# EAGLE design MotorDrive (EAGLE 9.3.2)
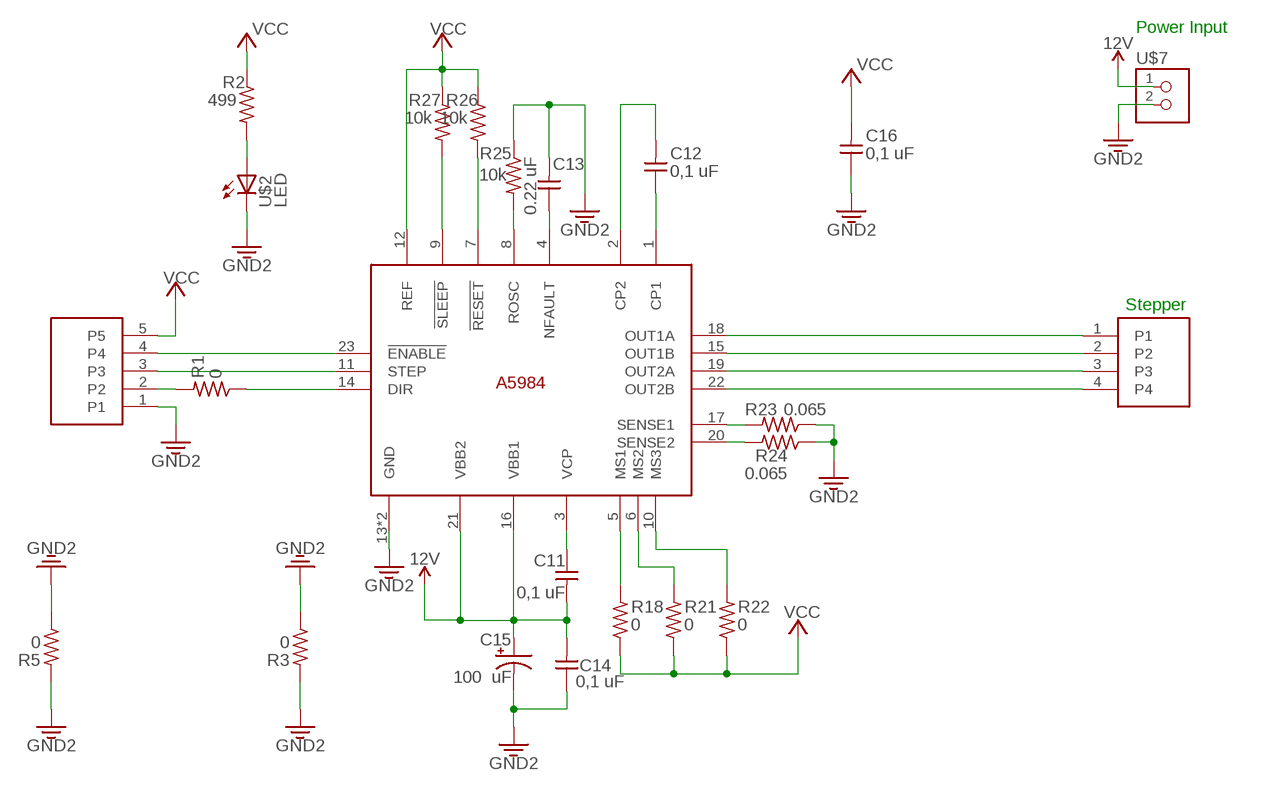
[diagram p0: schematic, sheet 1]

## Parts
C11  0,1 uF  CAP-UNPOLARIZED  [C1206]
C12  0,1 uF  CAP-UNPOLARIZED  [C1206]
C13  0.22 uF  CAP-UNPOLARIZED  [C1206]
C14  0,1 uF  CAP-UNPOLARIZED  [C1206]
C15  100 uF  CPOL-USE  [PANASONIC_E]
C16  0,1 uF  CAP-UNPOLARIZED  [C1206]
R1  0  RES-US1206  [R1206]
R2  499  RES-US1206  [R1206]
R3  0  RES-US1206  [R1206]
R5  0  RES-US1206  [R1206]
R18  0  RES-US1206  [R1206]
R21  0  RES-US1206  [R1206]
R22  0  RES-US1206  [R1206]
R23  0.065  RES-US1206  [R1206]
R24  0.065  RES-US1206  [R1206]
R25  10k  RES-US1206  [R1206]
R26  10k  RES-US1206  [R1206]
R27  10k  RES-US1206  [R1206]
U$1  HEADERPIN_X5  [1X05SMD]
U$2  LED  [LED1206]
U$7  HEADERPIN_X2  [1X02SMD]
U$19  A5984  [TSSOP24]
U$20  HEADERPIN_X4  [1X04SMD]

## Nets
12V: C11.2 C14.2 C15.+ U$7.1 U$19.16(VBB1) U$19.21(VBB2)
GND: C13.2 C14.1 C15.- C16.1 R3.1 R3.2 R5.1 R5.2 R23.1 R24.1 R25.1 U$1.1 U$2.2(C) U$7.2 U$19.13(GND) U$19.24(GND) ; supply symbol labelled GND2
N$1: R1.2 U$1.2
N$2: R2.2 U$2.1(A)
N$3: R1.1 U$19.14(DIR)
N$38: C12.1 U$19.1(CP1)
N$39: C12.2 U$19.2(CP2)
N$40: C11.1 U$19.3(VCP)
N$42: R18.2 U$19.5(MS1)
N$43: R21.2 U$19.6(MS2)
N$44: R22.2 U$19.10(MS3)
N$45: R23.2 U$19.17(SENSE1)
N$46: R24.2 U$19.20(SENSE2)
N$47: U$19.18(OUT1A) U$20.1
N$48: U$19.22(OUT2B) U$20.4
N$49: C13.1 U$19.4(NFAULT)
N$50: R27.2 U$19.9(!SLEEP)
N$51: R26.2 U$19.7(!RESET)
N$52: R25.2 U$19.8(ROSC)
N$53: U$19.15(OUT1B) U$20.2
N$54: U$19.19(OUT2A) U$20.3
N$59: U$1.3 U$19.11(STEP)
N$60: U$1.4 U$19.23(!ENABLE)
VCC: C16.2 R2.1 R18.1 R21.1 R22.1 R26.1 R27.1 U$1.5 U$19.12(REF)

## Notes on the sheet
- Power Input
- Stepper

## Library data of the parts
C11-C14 C16 = Fablab:CAP-UNPOLARIZED
C15 = rcl:CPOL-US: POLARIZED CAPACITOR, American symbol; SPICEPREFIX: C
R1-R3 R5 R18 R21-R27 = Fablab:RES-US: Resistor (US Symbol)
U$1 = Fablab:HEADERPIN_X5
U$2 = Fablab:LED: LED
U$7 = Fablab:HEADERPIN_X2
U$19 = MyAllegro:A5984
U$20 = Fablab:HEADERPIN_X4

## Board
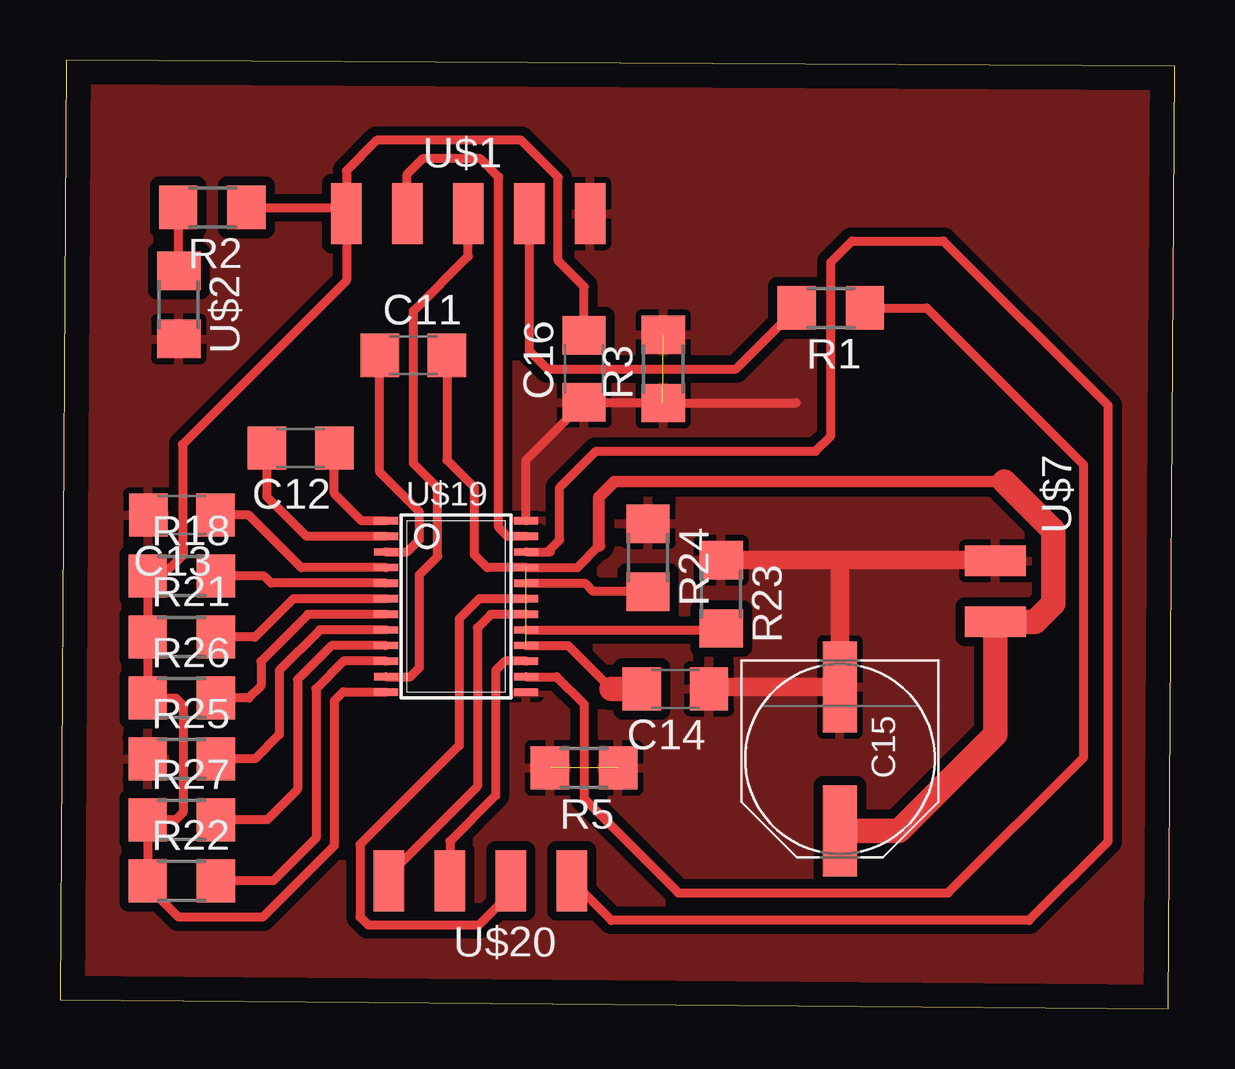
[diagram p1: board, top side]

Size 46.46 x 39.55 mm. Coordinates in mm from the lower left corner, seen from the top.
Outline: 0,0.38 46.21,0 46.46,39.29 0.25,39.55 0,0.38
Copper layers (1*16): Top 0.035mm / dielectric 1.5mm / Bottom 0.035mm
Design rules "default *": minimum track width 6mil, minimum drill 0.35mm, track to track 15mil, track to pad 15mil, pad to pad 15mil, via to via 15mil, smd to smd 6mil, copper to edge 40mil, drill to drill 6mil, minimum pad ring 10mil, minimum via ring 8mil, stop-mask expansion 4mil, vias tented up to drill 0mil, thermal gap 10mil

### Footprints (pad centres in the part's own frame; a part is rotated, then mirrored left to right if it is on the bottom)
C1206 = smd 1.6 x 1.8: 1 -1.4,0; 2 1.4,0
PANASONIC_E = smd 3.8 x 1.4: + 3,0; - -3,0
R1206 = smd 1.6 x 1.803: 1 -1.422,0; 2 1.422,0
1X05SMD = smd 2.54 x 1.27: 1 0,3.81; 2 0,1.27; 3 0,-1.27; 4 0,-3.81; 5 0,-6.35
LED1206 = smd 1.6 x 1.803: 1 -1.422,0; 2 1.422,0
1X02SMD = smd 2.54 x 1.27: 1 0,3.81; 2 0,1.27
TSSOP24 = smd 0.305 x 0.991: 1 -3.575,-2.918; 2 -2.925,-2.918; 3 -2.275,-2.918; 4 -1.625,-2.918; 5 -0.975,-2.918; 6 -0.325,-2.918; 7 0.325,-2.918; 8 0.975,-2.918; 9 1.625,-2.918; 10 2.275,-2.918; 11 2.925,-2.918; 12 3.575,-2.918; 13 3.575,2.918; 14 2.925,2.918; 15 2.275,2.918; 16 1.625,2.918; 17 0.975,2.918; 18 0.325,2.918; 19 -0.325,2.918; 20 -0.975,2.918; 21 -1.625,2.918; 22 -2.275,2.918; 23 -2.925,2.918; 24 -3.575,2.918
1X04SMD = smd 2.54 x 1.27: 1 0,3.81; 2 0,1.27; 3 0,-1.27; 4 0,-3.81

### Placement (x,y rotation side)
C11  14.73,27.23 0 top
C12  10.03,23.37 180 top
C13  5.08,20.57 180 top
C14  25.65,13.34 180 top
C15  32.51,10.41 270 top
C16  21.84,26.67 90 top
R1  32.13,29.21 180 top
R2  6.35,33.4 180 top
R3  25.15,26.67 90 top
R5  21.84,10.03 180 top
R18  5.08,18.03 0 top
R21  5.08,15.49 0 top
R22  5.08,5.33 0 top
R23  27.56,17.27 270 top
R24  24.51,18.8 270 top
R25  5.08,10.41 0 top
R26  5.08,12.95 0 top
R27  5.08,7.87 0 top
U$1  18.29,33.15 270 top
U$2  4.95,29.34 270 top
U$7  38.99,19.94 180 top
U$19  16.51,16.76 270 top
U$20  17.53,5.33 90 top

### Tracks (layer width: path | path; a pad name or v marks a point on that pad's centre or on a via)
12V  (1 unrouted)
  Top 0.381: U$19.16 21.18,15.14 22.99,13.34 | 22.48,19.3 21.56,18.39 U$19.21 17.81,18.39 17.27,18.92 17.27,21.72 16.13,22.86 C11.2 | C14.2 24.28,13.31
  Top 0.483: 23.11,21.97 39.37,21.97
  Top 0.508: 22.48,19.3 22.48,21.34 23.11,21.97
  Top 1.016: 22.99,13.34 C14.2 | C15.+ 34.97,7.41 38.99,11.43 U$7.1 40.64,16.13 41.4,16.89 41.4,19.94 39.37,21.97
GND  (2 unrouted)
  Top 0.381: U$19.24 19.43,22.88 21.82,25.27 C16.1 25.12,25.27 R3.1 30.68,25.25 | C14.1 27.13,13.41 | 38.96,18.69 U$7.2 | 32.51,18.57 32.38,18.69
  Top 0.762: 27.13,13.41 C15.- 32.51,18.57 | R23.1 32.38,18.69 38.96,18.69
  pour Top: 0.13,0.13 46.48,0.13 46.48,39.24 0.13,39.24
N$1
  Top 0.381: R1.2 28.17,26.67 20.32,26.67 19.56,27.43 U$1.2
N$2
  Top 0.381: R2.2 4.93,30.78 U$2.1
N$3
  Top 0.381: 34.1,29.76 R1.1 36.13,29.21 42.67,22.67 42.67,10.48 37.02,4.83 25.78,4.83 21.84,8.76 21.84,12.7 20.7,13.84 U$19.14
N$38
  Top 0.381: U$19.1 12.58,20.34 11.43,21.48 C12.1
N$39
  Top 0.381: U$19.2 10.28,19.69 8.63,21.34 C12.2
N$40
  Top 0.381: U$19.3 14.47,19.04 14.99,19.56 14.99,20.7 13.33,22.36 C11.1
N$42
  Top 0.381: U$19.5 8.8,17.74 8.51,18.03 R18.2
N$43
  Top 0.381: U$19.6 9.72,17.09 8.13,15.49 R21.2
N$44
  Top 0.381: R22.2 8.89,5.33 10.67,7.11 10.67,13.34 11.82,14.49 U$19.10
N$45
  Top 0.381: U$19.17 27.5,15.79 R23.2
N$46
  Top 0.381: U$19.20 21.89,17.74 22.23,17.4 24.49,17.4 R24.2
N$47
  Top 0.381: U$20.1 13.72,5.59 17.4,9.27 17.4,15.88 17.96,16.44 U$19.18
N$48
  Top 0.381: U$20.4 22.99,3.68 40.39,3.68 43.69,6.98 43.69,25.15 36.83,32 33.02,32 32.13,31.11 32.13,23.88 31.5,23.24 22.35,23.24 20.83,21.72 20.83,19.55 20.32,19.04 | U$19.22 20.32,19.04 | 20.32,19.04 20.44,19.04
N$49
  Top 0.381: U$19.4 10.06,18.39 7.87,20.57 C13.1
N$50
  Top 0.381: U$19.9 11.33,15.14 9.91,13.72 9.91,9.14 8.64,7.87 R27.2
N$51
  Top 0.381: U$19.7 10.34,16.44 8.38,14.48 8.38,13.46 7.87,12.95 R26.2
N$52
  Top 0.381: U$19.8 10.84,15.79 9.14,14.1 9.14,11.43 8.13,10.41 R25.2
N$53
  Top 0.381: U$19.15 18.55,14.49 18.16,14.1 18.16,8.89 16.26,6.98 U$20.2
N$54
  Top 0.381: U$19.19 17.47,17.09 16.64,16.26 16.64,10.97 12.51,6.84 12.51,3.83 12.84,3.49 17.46,3.49 18.8,4.83 U$20.3
N$59
  Top 0.381: U$19.11 14.6,13.84 14.99,14.22 14.99,18.1 15.75,18.86 15.75,21.72 14.73,22.73 14.73,29.08 17.02,31.37 U$1.3
N$60
  Top 0.381: U$1.4 14.48,34.8 15.11,35.43 17.53,35.43 18.29,34.67 18.29,20.07 18.66,19.69 U$19.23
VCC
  Top 0.381: U$19.12 11.83,13.19 11.81,13.21 11.43,12.83 11.43,6.8 8.44,3.81 4.95,3.81 3.66,5.1 R22.1 R27.1 4.83,7.87 5.13,8.18 5.13,12.65 4.83,12.95 R26.1 R21.1 R18.1 4.24,18.03 5.13,18.92 5.13,19.41 5.11,19.44 5.11,23.52 11.94,30.35 U$1.5 | C16.2 21.84,30.1 20.77,31.18 20.77,34.65 19.22,36.2 13.21,36.2 11.94,34.93 U$1.5 | R2.1 11.68,33.4 U$1.5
